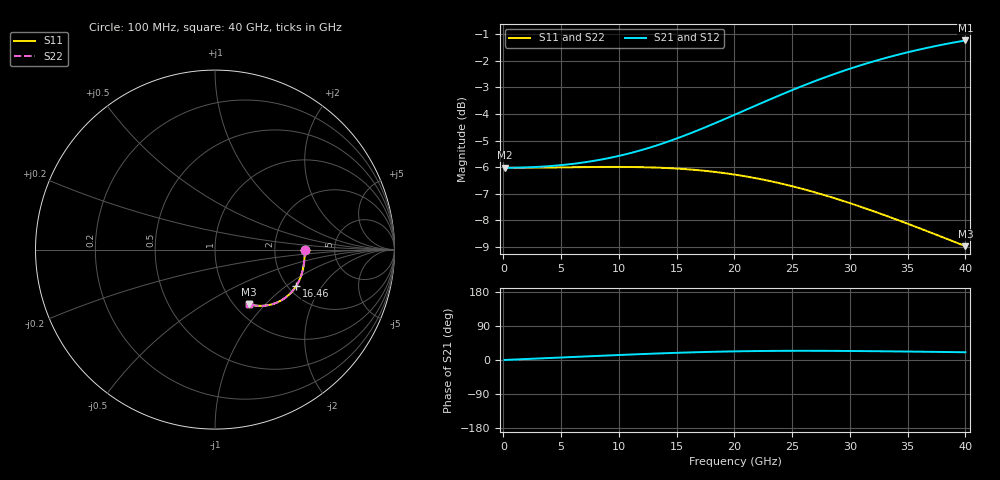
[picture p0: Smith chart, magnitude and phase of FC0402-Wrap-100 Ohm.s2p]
!Vishay Thin-Film
!FC Family
!Case Size 0402
!Assembly Style Full Wrap SMT
!10/21/2015
!thinfilm@vishay.com
# GHz S MA R 50
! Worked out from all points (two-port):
!   101 points, 100 MHz to 40 GHz, reference 50 ohm
!   highest |S21| = -1.23 dB at 40 GHz (marker M1); lowest = -6.0 dB at 100 MHz (marker M2)
!   |S21| within 3 dB of the highest: 18.93 GHz to end of sweep
!   lowest |S11| = -9.0 dB at 40 GHz (marker M3), VSWR 2.11, Z = 58 - j40.2 ohm
!   |S11| at or under -10 dB: nowhere
!   |S22| runs from -9.0 to -6.0 dB; largest |S21 - S12| = 0
!   S11 on the Smith chart (normalised r, x): 100 MHz: 3.00, -0.01; 16.46 GHz: 2.21, -1.19; 40 GHz: 1.16, -0.80
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0.1  0.5 -0.1  0.5 0.1  0.5 0.1  0.5 -0.1
2.095  0.5002 -2.8  0.501 2.8  0.501 2.8  0.5002 -2.8
3.691  0.5005 -4.9  0.5031 4.9  0.5031 4.9  0.5005 -4.9
6.883  0.5015 -9.3  0.5115 9.1  0.5115 9.1  0.5015 -9.3
8.878  0.5019 -12.2  0.5202 11.7  0.5202 11.7  0.5019 -12.2
10.474  0.5018 -14.5  0.5294 13.8  0.5294 13.8  0.5018 -14.5
12.07  0.5013 -17.0  0.5408 15.7  0.5408 15.7  0.5013 -17.0
13.666  0.5 -19.5  0.5545 17.5  0.5545 17.5  0.5 -19.5
15.262  0.4979 -22.1  0.5704 19.2  0.5704 19.2  0.4979 -22.1
16.459  0.4957 -24.1  0.5837 20.3  0.5837 20.3  0.4957 -24.1
18.055  0.4918 -26.8  0.6031 21.6  0.6031 21.6  0.4918 -26.8
20.05  0.4854 -30.2  0.6295 22.8  0.6295 22.8  0.4854 -30.2
22.045  0.4771 -33.5  0.6575 23.6  0.6575 23.6  0.4771 -33.5
23.641  0.4692 -36.2  0.6805 24.0  0.6805 24.0  0.4692 -36.2
25.237  0.4602 -38.8  0.7033 24.2  0.7033 24.2  0.4602 -38.8
26.833  0.4504 -41.4  0.7258 24.2  0.7258 24.2  0.4504 -41.4
28.429  0.4399 -43.8  0.7475 24.1  0.7475 24.1  0.4399 -43.8
30.025  0.4288 -46.2  0.7682 23.8  0.7682 23.8  0.4288 -46.2
31.621  0.4174 -48.4  0.7877 23.4  0.7877 23.4  0.4174 -48.4
33.616  0.4027 -51.1  0.8102 22.8  0.8102 22.8  0.4027 -51.1
36.808  0.3791 -55.0  0.8417 21.6  0.8417 21.6  0.3791 -55.0
40  0.3561 -58.4  0.8679 20.4  0.8679 20.4  0.3561 -58.4
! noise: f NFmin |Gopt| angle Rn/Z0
0.1  1.83e-07  1  -1.242e-17  2
4.489  -7.232e-15  1  -4.019e-15  1.942
8.878  2.893e-15  1  -8.538e-07  1.764
13.27  1.929e-15  1  5.347e-15  1.47
17.66  -2.411e-15  1  -1.479e-06  1.116
22.05  -1.929e-15  1  -7.014e-15  0.7866
26.43  -4.822e-16  1  8.642e-15  0.5321
30.82  4.607e-08  1  2.583e-14  0.3559
35.21  3.106e-08  1  -2.425e-14  0.24
40  2.061e-08  1  -1.657e-14  0.1592
